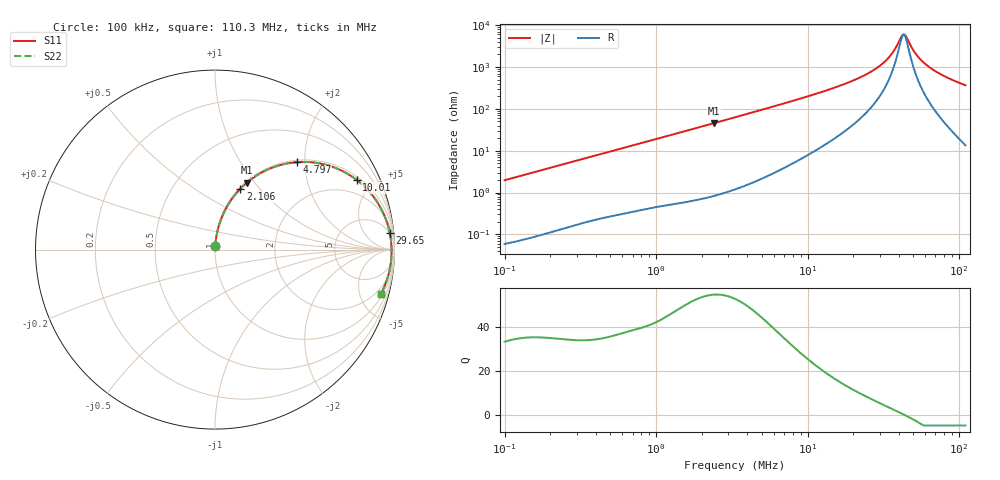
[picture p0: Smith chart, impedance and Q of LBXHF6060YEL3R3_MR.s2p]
! LBXHF6060YEL3R3_MR  S-PARAMETER MODEL  ( General Type )
! Model Generated by TAIYO YUDEN Corporation (http://www.ty-top.com)
! Version 1.0
! TAIYO YUDEN Control No. 201201NI43SB-FBB
! Copyright(c) 2020 TAIYO YUDEN CO.,LTD. All Rights Reserved.
! Product Description (link to TY-COMPAS)
! https://ds.yuden.co.jp/TYCOMPAS/or/detail?pn=LBXHF6060YEL3R3MMR&u=M
! Products Name : Inductors
! Characteristics :
!  Inductance : 3.3 uH , SRF(min) : 32 MHz , DC Resistance(max) : 0.0276 Ohm
!  Rated Current : Saturation :7000 mA , Temp Rise : 2500 mA
!  Case Size : 6.0 x 6.0 / 0.236 x 0.236 [mm/inch] , Thickness : 4.5 / 0.177 [mm/inch]
!  (Conditions: Temperature = 25 degC , DC Bias Current/Voltage = 0A / 0V)
! External Node Assignments :
!  1  o---GGG---o  2
! GND o---------o GND
! Frequency Range : 0.1MHz  -  110.285862MHz  [ 402 STEP ]
# MHz S RI R 50
! Freq[MHz].  S11 Real  S11 Imag  S21 Real  S21 Imag  S12 Real  S12 Imag  S22 Real  S22 Imag
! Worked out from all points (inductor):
!   401 points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, 100 kHz to 110.3 MHz, reference 50 ohm
!   read as one part in series: L = 3.13 uH near 103.6 kHz
!   highest Q = 54.9 at 2.423 MHz (marker M1), where L = 3 uH
!   self-resonance near 42.83 MHz
!   S11 on the Smith chart (normalised r, x): 100 kHz: 1.00, +0.04; 2.106 MHz: 1.01, +0.79; 4.797 MHz: 1.04, +1.82; 10.01 MHz: 1.16, +3.97; 29.65 MHz: 5, +20; 110.3 MHz: 1.27, -7.32
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0.1  0.000977 0.0197  0.999 -0.0197  0.999 -0.0197  0.000977 0.0197
0.323312  0.00572 0.0621  0.9943 -0.0621  0.9943 -0.0621  0.00572 0.0621
1.045308  0.0418 0.1889  0.9582 -0.1889  0.9582 -0.1889  0.0418 0.1889
2.106183  0.1409 0.3388  0.8591 -0.3388  0.8591 -0.3388  0.1409 0.3388
2.422962  0.1773 0.3729  0.8227 -0.3729  0.8227 -0.3729  0.1773 0.3729
3.320932  0.2864 0.4427  0.7136 -0.4427  0.7136 -0.4427  0.2864 0.4427
4.797248  0.4552 0.4871  0.5448 -0.4871  0.5448 -0.4871  0.4552 0.4871
6.809547  0.6287 0.4694  0.3713 -0.4694  0.3713 -0.4694  0.6287 0.4694
10.01052  0.7884 0.3892  0.2116 -0.3892  0.2116 -0.3892  0.7884 0.3892
10.73698  0.8116 0.3705  0.1884 -0.3705  0.1884 -0.3705  0.8116 0.3705
19.81995  0.941 0.1962  0.059 -0.1962  0.059 -0.1962  0.941 0.1962
24.88768  0.9632 0.1355  0.0368 -0.1355  0.0368 -0.1355  0.9632 0.1355
29.65155  0.9741 0.0911  0.0259 -0.0911  0.0259 -0.0911  0.9741 0.0911
34.71395  0.9802 0.0525  0.0198 -0.0525  0.0198 -0.0525  0.9802 0.0525
37.89096  0.9823 0.0314  0.0177 -0.0314  0.0177 -0.0314  0.9823 0.0314
41.35872  0.9835 0.0103  0.0165 -0.0103  0.0165 -0.0103  0.9835 0.0103
43.58991  0.9838 -0.00226  0.0162 0.00226  0.0162 0.00226  0.9838 -0.00226
45.14385  0.9838 -0.0107  0.0162 0.0107  0.0162 0.0107  0.9838 -0.0107
51.93366  0.9825 -0.0446  0.0175 0.0446  0.0175 0.0446  0.9825 -0.0446
60.80029  0.9782 -0.0838  0.0218 0.0838  0.0218 0.0838  0.9782 -0.0838
79.06789  0.963 -0.1529  0.037 0.1529  0.037 0.1529  0.963 -0.1529
110.2859  0.9228 -0.2492  0.0772 0.2492  0.0772 0.2492  0.9228 -0.2492
